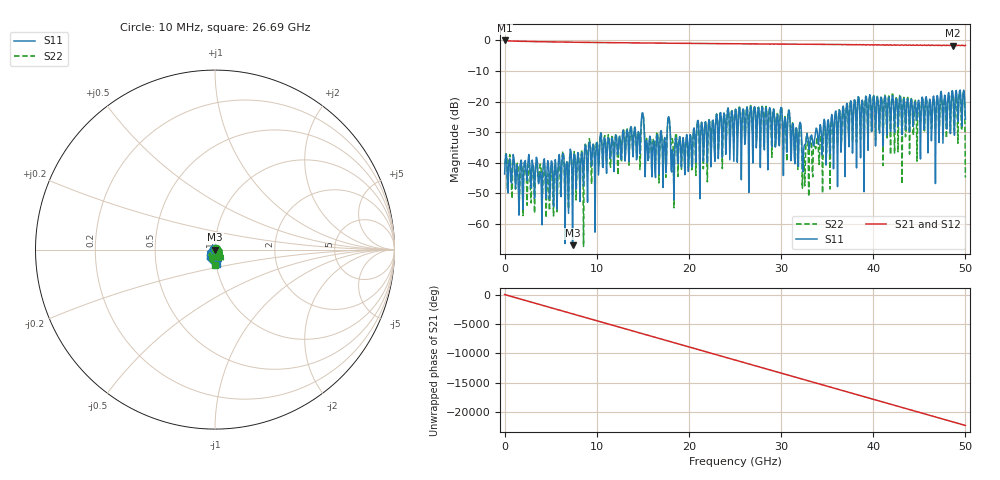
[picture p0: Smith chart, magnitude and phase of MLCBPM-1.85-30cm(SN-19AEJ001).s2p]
!Keysight Technologies,N5225A,MY51451228,A.10.40.14
!Date: Monday, March 22, 2021 13:48:12
!Correction: S11(Full 2 Port(1,3))
!S31(Full 2 Port(1,3))
!S13(Full 2 Port(1,3))
!S33(Full 2 Port(1,3))
!S2P File: Measurements: S11, S31, S13, S33:
# Hz S  dB  R 50
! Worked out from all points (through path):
!   801 points, 10 MHz to 50 GHz, reference 50 ohm
!   highest |S21| = -0.02 dB at 10 MHz (marker M1); lowest = -1.7 dB at 48.63 GHz (marker M2)
!   group delay of S21, straight-line fit = 1.24 ns
!   lowest |S11| = -67.0 dB at 7.384 GHz (marker M3), VSWR 1.00, Z = 50 + j0.041 ohm
!   |S11| at or under -10 dB: start of sweep to end of sweep
!   |S22| runs from -67.3 to -16.6 dB; largest |S21 - S12| = 0.014
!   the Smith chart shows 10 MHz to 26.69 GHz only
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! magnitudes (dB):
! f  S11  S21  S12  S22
! 10 MHz  -43.7  0.0  0.0  -40.5
! 4.697 GHz  -39.3  -0.5  -0.5  -43.6
! 7.384 GHz  -67.0  -0.6  -0.6  -50.4
! 8.383 GHz  -36.7  -0.6  -0.6  -35.8
! 9.008 GHz  -52.9  -0.7  -0.6  -43.3
! 14.51 GHz  -29.8  -0.8  -0.8  -29.9
! 15.07 GHz  -25.1  -0.8  -0.8  -24.9
! 16.13 GHz  -33.6  -0.9  -0.9  -32.4
! 16.69 GHz  -36.2  -0.9  -0.9  -35.3
! 17.38 GHz  -31.7  -0.9  -0.9  -32.1
! 17.82 GHz  -24.9  -0.9  -0.9  -25.0
! 18.26 GHz  -36.3  -0.9  -0.9  -32.8
! 25 GHz  -23.6  -1.1  -1.1  -23.4
! 28.13 GHz  -32.8  -1.2  -1.2  -29.5
! 31 GHz  -28.7  -1.2  -1.2  -28.5
! 32.44 GHz  -36.3  -1.3  -1.3  -36.6
! 33.38 GHz  -31.9  -1.3  -1.3  -42.2
! 37.38 GHz  -34.8  -1.4  -1.4  -30.3
! 41.69 GHz  -18.5  -1.6  -1.6  -18.1
! 48.63 GHz  -16.8  -1.7  -1.7  -17.8
! 49.63 GHz  -28.0  -1.6  -1.6  -28.9
! 50 GHz  -25.7  -1.6  -1.6  -44.9
